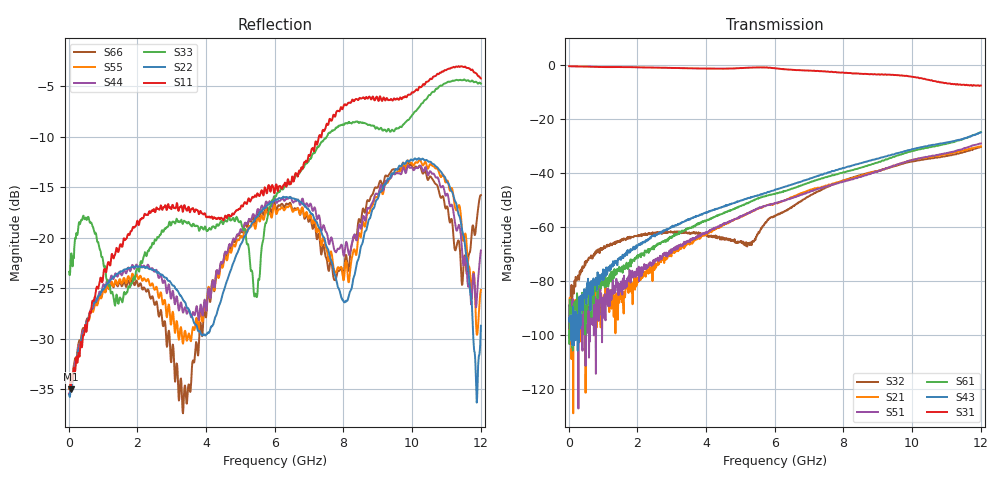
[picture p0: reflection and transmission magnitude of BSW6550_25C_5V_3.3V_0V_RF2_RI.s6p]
! Agilent Technologies	N5230C	MY49001333	A.09.33.09
!	Test time	=	2026-05-06 10:00
!	Product	=	BSW6550
!	Temp	=	25C
!	VDD	=	5
!	Control_High	=	3.3
!	Control_Low	=	0
!	Logic	=	RF2
!	Port1	=	RFC
!	Port2	=	RF1
!	Port3	=	RF2
!	Port4	=	RF3
!	Port5	=	RF4
!	Port6	=	RF5
!	V1	=	3.3 / 0
!	V2	=	3.3 / 0
!	V3	=	3.3 / 0
!S6P File: Measurements: <S11,S12,S13,S14,S15,S16>,
!<S21,S22,S23,S24,S25,S26>,
!<S31,S32,S33,S34,S35,S36>,
!<S41,S42,S43,S44,S45,S46>,
!<S51,S52,S53,S54,S55,S56>,
!<S61,S62,S63,S64,S65,S66>;
# HZ S RI R 50
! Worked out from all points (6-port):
!   1201 points, 10 MHz to 12.01 GHz, reference 50 ohm
!   strongest paths, dB at 10 MHz, 3.01 GHz, 6.01 GHz, 9.01 GHz, 12.01 GHz:
!     S31: -0.5, -1.2, -1.3, -3.5, -7.7
!     S43: -94.0, -60.2, -46.3, -34.7, -25.0
!     S61: -103.3, -63.6, -47.9, -36.2, -25.0
!     S51: -97.4, -69.4, -51.4, -39.5, -29.2
!     S21: -94.6, -69.7, -51.3, -39.5, -30.2
!     S32: -94.9, -61.9, -55.9, -39.3, -30.4
!   lowest |S11| = -35.1 dB at 60 MHz (marker M1), VSWR 1.04, Z = 51.8 - j0.268 ohm
!   |S11| at or under -10 dB: start of sweep to 7.288 GHz; 7.345041 GHz to 7.361897 GHz (16.86 MHz wide, 0.229 % of centre)
